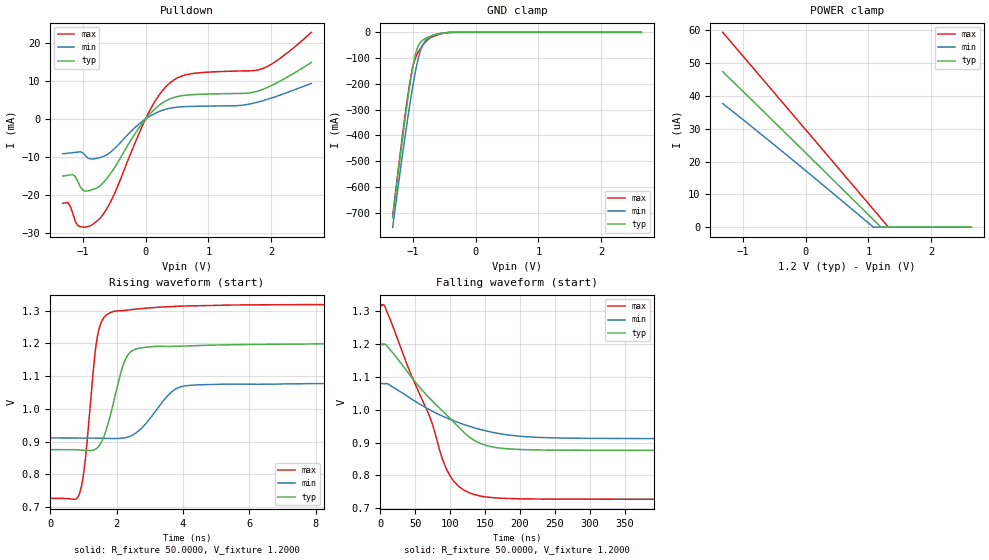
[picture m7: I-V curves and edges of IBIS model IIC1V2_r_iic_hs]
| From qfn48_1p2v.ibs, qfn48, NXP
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[Model] IIC1V2_r_iic_hs
|   Model IIC1V2_r_iic_hs
| This model was characterised for following simulation conditions:
| External (pad) voltage:
|   - Typ: 1.2V,   - Min: 1.08V,   - Max: 1.32V
| Library cells for typ/min/max conditions are connected as defined below:
|  IO - External Pad
|  A - Core Input
|  EN - Output Buffer Enable
|  BOOST - vdde
|  ECS - gnd
|  EGP - gnd
|  ENZI - vdd
|  EPD - vdd
|  EPUN - gnd
|  ZI - NC
|  ZIF - NC
|  gnd - gnd
|  gnde - gnde
|  vdd - vdd
|  vdde - vdde
| All other pins connected to ground
Model_type I/O_open_drain
Polarity   Non-Inverting
Enable   Active-Low
Vinl =   0.5400V
Vinh =   1.2600V
Vmeas =  0.9000V
Cref =   0.0F
Rref =   1.0000k
Vref =   1.2000V
C_comp   3.6168pF   3.4770pF   3.7425pF
|C_comp_pullup   0.9409pF   0.9008pF   0.9551pF
|C_comp_pulldown   2.3238pF   2.4763pF   2.1787pF
[Model Spec]
| variable   typ   min   max
Vinh   0.3600V   0.3240V   0.3960V
Vinl   0.8400V   0.7560V   0.9240V
Vmeas   0.6000V   0.5400V   0.6600V
Vref   1.2000V   1.0800V   1.3200V
Cref   0.0F   0.0F   0.0F
Rref   1.0000k   1.0000k   1.0000k
[Temperature Range]   25.0000   0.1250k   -40.0000
[Voltage Range]   1.2000V   1.0800V   1.3200V
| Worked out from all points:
|   slope of the pulldown table from 0 to 0.18 V, typ, clamps not added: 58.3 ohm
|   GND clamp passes 1 mA (typ) near -0.45 V on its own axis
|   rising waveform, R_fixture 50.0000, V_fixture 1.2000: 20-80 % time 501ps typ, 802ps min, 332ps max; typ from 0.876 V to 1.2 V
|   falling waveform, R_fixture 50.0000, V_fixture 1.2000: 20-80 % time 83.3ns typ, 99ns min, 62.6ns max; typ from 1.2 V to 0.876 V
[Pulldown]
|Voltage   I(typ)   I(min)   I(max)
-1.32V    -14.96mA   -9.099mA   -22.09mA
-1.24V    -14.75mA   -8.982mA   -21.89mA
-1.16V    -14.56mA   -8.83mA    -24.7mA
-1.04V    -17.82mA   -8.609mA   -28.21mA
-920mV    -18.88mA   -10.21mA   -28.21mA
-720mV    -17.44mA   -10.07mA   -25.94mA
-520mV    -13.41mA   -8.157mA   -20.44mA
80mV      1.521mA    840uA      2.628mA
440mV     5.569mA    2.951mA    10.1mA
760mV     6.377mA    3.307mA    11.92mA
1.84V     7.592mA    4.649mA    13.07mA
2.64V     14.79mA    9.287mA    22.7mA
[GND_clamp]
|Voltage   I(typ)   I(min)   I(max)
-1.32V    -720.7mA   -756.5mA   -713.8mA
-1.12V    -330.9mA   -399.5mA   -316.8mA
-1.04V    -192.4mA   -269.2mA   -184.4mA
-1V       -133.6mA   -209.3mA   -133.5mA
-960mV    -86.74mA   -154.7mA   -99.46mA
-920mV    -55.69mA   -108.2mA   -79.02mA
-880mV    -39.02mA   -72.35mA   -63.71mA
-840mV    -29.9mA    -48mA      -50.26mA
-760mV    -18.93mA   -23.39mA   -28.32mA
-640mV    -9.22mA    -8.628mA   -12.73mA
-400mV    -335.3uA   -402.3uA   -442.6uA
2.64V     0A         0A         0A
[POWER_clamp]
|Voltage   I(typ)   I(min)   I(max)
-1.32V    47.4uA     37.67uA    59.39uA
-280mV    27.94uA    21.65uA    36.04uA
1.08V     2.274uA    0A         5.413uA
1.2V      0A         0A         2.707uA
1.32V     0A         0A         0A
2.64V     0A         0A         0A
[Ramp]
| variable   typ   min   max
dV/dt_r  0.1938/0.5014n   0.1006/0.8017n   0.3548/0.3320n
dV/dt_f  0.1938/83.2452n   0.1006/98.9100n   0.3548/62.5577n
R_load = 50.0000
[Rising Waveform]
R_fixture= 50.0000
V_fixture= 1.2000
V_fixture_min= 1.0800
V_fixture_max= 1.3200
|time   V(typ)   V(min)   V(max)
0s        875.8mV    911.4mV    727.2mV
889.8ps   874.9mV    911.6mV    744.3mV
1.063ns   873.7mV    911.5mV    850.9mV
1.382ns   878.1mV    911mV      1.196V
1.663ns   928.5mV    910.2mV    1.284V
2.172ns   1.125V     910.6mV    1.3V
2.484ns   1.178V     920.4mV    1.303V
3.862ns   1.191V     1.065V     1.313V
6.246ns   1.197V     1.075V     1.318V
1us       1.199V     1.079V     1.319V
[Falling Waveform]
R_fixture= 50.0000
V_fixture= 1.2000
V_fixture_min= 1.0800
V_fixture_max= 1.3200
|time   V(typ)   V(min)   V(max)
0s        1.199V     1.079V     1.319V
6.434ns   1.199V     1.078V     1.315V
43.44ns   1.102V     1.034V     1.11V
71.42ns   1.033V     998.8mV    974.9mV
95.84ns   981.8mV    974mV      814.3mV
114.6ns   941.6mV    958.5mV    762.6mV
138.3ns   902.1mV    942.4mV    739.5mV
175.9ns   881.9mV    925.1mV    730.2mV
271.8ns   876.6mV    913.1mV    727.7mV
1us       875.9mV    911.5mV    727.2mV
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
